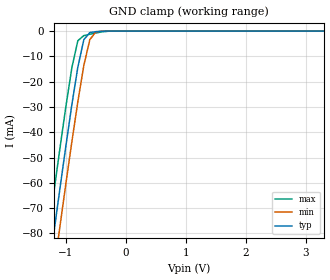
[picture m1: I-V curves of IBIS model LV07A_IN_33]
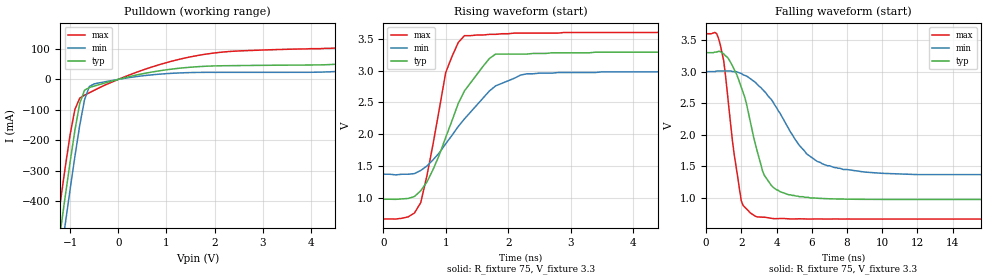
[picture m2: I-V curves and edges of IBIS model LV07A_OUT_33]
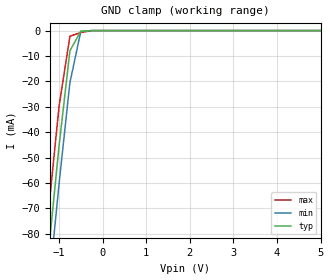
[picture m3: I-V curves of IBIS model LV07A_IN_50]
| TEXAS INSTRUMENTS INCORPORATED
| Standard Linear and Logic Group
| IBIS Model of SN74LV07A
| HEX BUFFER with OPEN DRAIN OUTPUTS
| SOIC 14-pin (D), SOP 14-pin (NS), SSOP 14-pin (DB), TSSOP 14-pin (PW)
| and TVSOP 14-pin (DGV) Package
[IBIS Ver]   3.2
[Comment Char]  |_char
[File Name]   sn74lv07a.ibs
[File Rev]   1.1
[Date]   July 27, 2004
[Source]   Data created from HSPICE simulations at TI-SLL.
[Notes]   The following is an IBIS list for the LV07A.
|   Please contact sllibis@ti.com with questions and
|   comments concerning SLL IBIS models.
   - FILE REV HISTORY
   - 1.1 Release IBIS file on 07/27/04
[Disclaimer] Property of Texas Instruments Incorporated.  Unauthorized
   reproduction and/or distribution is strictly prohibited.
   This product is protected under copyright law.
   Created  2004, (C) Copyright  2004, Texas Instruments
   Incorporated, All Rights Reserved
   UNLESS THERE IS A SIGNED, WRITTEN AGREEMENT TO THE
   CONTRARY, TEXAS INSTRUMENTS (TI) IS PROVIDING THE IBIS
   MODELS  AND WITHOUT ANY WARRANTY, EXPRESSED OR
   IMPLIED.  TI assumes no liability for:
   1) the accuracy of the IBIS models provided to your
   company;
   2) the proper functioning of these IBIS Models in your
   design or for any resulting applications; or
   3) infringement of patents, copyrights or intellectual
   property rights resulting from your use of these IBIS
   models.
   TI provides IBIS Models as a service to our customers.
   You and your company shall not distribute, sell or give
   these models to anyone else without prior written
   permission from TI.
   TI reserves the right to make changes to our products or
   to discontinue any semiconductor product or service
   without notice, and advises our customers to obtain the
   latest version of relevant information to verify, before
   placing orders, that the information being relied on is
   current.
   Please be aware that your receipt and use of the IBIS
   information provided shall serve as acceptance of these
   terms and conditions.  If you do not accept these terms,
   you should return or destroy the IBIS models and any
   other accompanying information immediately.
|   Component LV07A_D
[Component]   LV07A_D
[Manufacturer]  Texas Instruments, Inc.
[Package]
|   typ   min   max
R_pkg   0.031   0.028   0.034
L_pkg   3.109nH   2.462nH   3.889nH
C_pkg   0.473pF   0.363pF   0.628pF
[Pin]   signal_name   model_name   R_pin   L_pin   C_pin
1   1A   LV07A_IN   0.033   3.854nH   0.622pF
2   1Y   LV07A_OUT   0.032   3.188nH   0.473pF
3   2A   LV07A_IN   0.028   2.462nH   0.377pF
4   2Y   LV07A_OUT   0.031   2.596nH   0.363pF
5   3A   LV07A_IN   0.028   2.521nH   0.372pF
6   3Y   LV07A_OUT   0.034   3.250nH   0.476pF
7   GND   GND   0.034   3.889nH   0.628pF
8   4Y   LV07A_OUT   0.034   3.889nH   0.628pF
9   4A   LV07A_IN   0.034   3.250nH   0.476pF
10   5Y   LV07A_OUT   0.028   2.521nH   0.372pF
11   5A   LV07A_IN   0.031   2.596nH   0.364pF
12   6Y   LV07A_OUT   0.028   2.462nH   0.377pF
13   6A   LV07A_IN   0.032   3.188nH   0.473pF
14   VCC   POWER   0.033   3.854nH   0.622pF
|   Component LV07A_NS
[Component]   LV07A_NS
[Manufacturer]  Texas Instruments, Inc.
[Package]
|   typ   min   max
R_pkg   0.045   0.039   0.054
L_pkg   3.796nH   2.561nH   4.952nH
C_pkg   0.528pF   0.288pF   0.710pF
[Pin]   signal_name   model_name   R_pin   L_pin   C_pin
1   1A   LV07A_IN   0.047   4.867nH   0.706pF
2   1Y   LV07A_OUT   0.051   4.083nH   0.592pF
3   2A   LV07A_IN   0.041   2.915nH   0.376pF
4   2Y   LV07A_OUT   0.039   2.561nH   0.288pF
5   3A   LV07A_IN   0.041   3.101nH   0.430pF
6   3Y   LV07A_OUT   0.047   4.047nH   0.589pF
7   GND   GND   0.051   4.909nH   0.700pF
8   4Y   LV07A_OUT   0.045   4.784nH   0.694pF
9   4A   LV07A_IN   0.054   4.176nH   0.597pF
10   4Y   LV07A_OUT   0.039   3.287nH   0.449pF
11   5A   LV07A_IN   0.039   2.586nH   0.294pF
12   6Y   LV07A_OUT   0.040   2.802nH   0.371pF
13   6A   LV07A_IN   0.049   4.080nH   0.593pF
14   VCC   POWER   0.052   4.952nH   0.710pF
|   Component LV07A_DB
[Component]   LV07A_DB
[Manufacturer]  Texas Instruments, Inc.
[Package]
|   typ   min   max
R_pkg   0.044   0.041   0.046
L_pkg   3.551nH   3.258nH   3.927nH
C_pkg   0.402pF   0.360pF   0.421pF
[Pin]   signal_name   model_name   R_pin   L_pin   C_pin
1   1A   LV07A_IN   0.046   3.927nH   0.408pF
2   1Y   LV07A_OUT   0.044   3.587nH   0.421pF
3   2A   LV07A_IN   0.041   3.289nH   0.398pF
4   2Y   LV07A_OUT   0.042   3.258nH   0.360pF
5   3A   LV07A_IN   0.041   3.286nH   0.403pF
6   3Y   LV07A_OUT   0.044   3.586nH   0.421pF
7   GND   GND   0.046   3.927nH   0.408pF
8   4Y   LV07A_OUT   0.046   3.927nH   0.408pF
9   4A   LV07A_IN   0.044   3.586nH   0.421pF
10   5Y   LV07A_OUT   0.041   3.286nH   0.403pF
11   5A   LV07A_IN   0.043   3.258nH   0.360pF
12   6Y   LV07A_OUT   0.041   3.289nH   0.398pF
13   6A   LV07A_IN   0.044   3.587nH   0.421pF
14   VCC   POWER   0.046   3.927nH   0.408pF
|   Component LV07A_PW
[Component]   LV07A_PW
[Manufacturer]  Texas Instruments, Inc.
[Package]
|   typ   min   max
R_pkg   0.032   0.029   0.035
L_pkg   2.378nH   2.170nH   2.680nH
C_pkg   0.314pF   0.270pF   0.335pF
[Pin]   signal_name   model_name   R_pin   L_pin   C_pin
1   1A   LV07A_IN   0.033   2.618nH   0.330pF
2   1Y   LV07A_OUT   0.031   2.313nH   0.317pF
3   2A   LV07A_IN   0.030   2.310nH   0.314pF
4   2Y   LV07A_OUT   0.031   2.173nH   0.272pF
5   3A   LV07A_IN   0.030   2.204nH   0.309pF
6   3Y   LV07A_OUT   0.032   2.315nH   0.317pF
7   GND   GND   0.035   2.680nH   0.335pF
8   4Y   LV07A_OUT   0.033   2.640nH   0.333pF
9   4A   LV07A_IN   0.034   2.347nH   0.319pF
10   5Y   LV07A_OUT   0.029   2.277nH   0.313pF
11   5A   LV07A_IN   0.031   2.170nH   0.270pF
12   6Y   LV07A_OUT   0.031   2.244nH   0.311pF
13   6A   LV07A_IN   0.033   2.343nH   0.321pF
14   VCC   POWER   0.035   2.657nH   0.332pF
|   Component LV07A_DGV
[Component]   LV07A_DGV
[Manufacturer]  Texas Instruments, Inc.
[Package]
|   typ   min   max
R_pkg   0.035   0.020   0.045
L_pkg   2.499nH   2.077nH   2.966nH
C_pkg   0.361pF   0.305pF   0.416pF
[Pin]   signal_name   model_name   R_pin   L_pin   C_pin
1   1A   LV07A_IN   0.027   2.717nH   0.373pF
2   1Y   LV07A_OUT   0.037   2.434nH   0.398pF
3   2A   LV07A_IN   0.034   2.200nH   0.316pF
4   2Y   LV07A_OUT   0.020   2.077nH   0.309pF
5   3A   LV07A_IN   0.030   2.147nH   0.305pF
6   3Y   LV07A_OUT   0.042   2.580nH   0.408pF
7   GND   GND   0.039   2.921nH   0.385pF
8   4Y   LV07A_OUT   0.033   2.841nH   0.380pF
9   4A   LV07A_IN   0.042   2.611nH   0.410pF
10   5Y   LV07A_OUT   0.038   2.331nH   0.329pF
11   5A   LV07A_IN   0.026   2.223nH   0.319pF
12   6Y   LV07A_OUT   0.034   2.259nH   0.313pF
13   6A   LV07A_IN   0.045   2.681nH   0.416pF
14   VCC   POWER   0.042   2.966nH   0.386pF
[Model Selector]   LV07A_IN
LV07A_IN_33   3.3-V Vcc Input Model
LV07A_IN_50   5.0-V Vcc Input Model
[Model Selector]   LV07A_OUT
LV07A_OUT_33   3.3-V Vcc Output Model
LV07A_OUT_50   5.0-V Vcc Output Model
| Models and submodels in the file (4): LV07A_IN_33 (Input), LV07A_OUT_33 (Open_drain), LV07A_IN_50 (Input), LV07A_OUT_50 (Open_drain)
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|   Model LV07A_IN_33
[Model]   LV07A_IN_33
Model_type  Input
Polarity   Non-Inverting
Vinl = 0.99
Vinh = 2.31
| variable   typ   min   max
C_comp   1.24pf   0.94pf   1.54pf
[Temperature Range]   25   85   -40
[Voltage Range]   3.3   3.0   3.6
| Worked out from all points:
|   GND clamp passes 1 mA (typ) near -0.61 V on its own axis
[GND Clamp]
|   Voltage   I(typ)   I(min)   I(max)
-3.3V     -460mA     -475mA     -445mA
-1.3V     -97.5mA    -113mA     -81.5mA
-1.2V     -79.9mA    -95mA      -63.9mA
-1.1V     -62.6mA    -77.6mA    -46.7mA
-1V       -45.6mA    -60.5mA    -30mA
-900mV    -29.2mA    -43.9mA    -14.6mA
-800mV    -14.3mA    -28mA      -3.81mA
-700mV    -3.42mA    -13.6mA    -1.78mA
-600mV    -581uA     -3.4mA     -1.25mA
-500mV    -233uA     -353uA     -759uA
-400mV    -58.1uA    -21.9uA    -324uA
3.3V      1.9nA      2.34nA     1.69nA
|   Model LV07A_OUT_33
[Model]   LV07A_OUT_33
Model_type  Open_drain
Polarity   Non-Inverting
Vmeas = 1.65v
Cref = 15pf
| variable   typ   min   max
C_comp   4.62pf   3.47pf   5.77pf
[Temperature Range]   25   85   -40
[Voltage Range]   3.3   3.0   3.6
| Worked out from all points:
|   slope of the pulldown table from 0 to 0.495 V, typ, clamps not added: 27.3 ohm
|   falling waveform, R_fixture 75, V_fixture 3.3: 20-80 % time 1.3ns typ, 2.37ns min, 767ps max; typ from 3.3 V to 0.976 V
|   rising waveform, R_fixture 75, V_fixture 3.3: 20-80 % time 624ps typ, 807ps min, 340ps max; typ from 0.976 V to 3.3 V
[Pulldown]
|   Voltage   I(typ)   I(min)   I(max)
-3.3V     -3.04A     -3.13A     -2.95A
-1.3V     -615mA     -707mA     -518mA
-1.2V     -498mA     -591mA     -401mA
-1.1V     -383mA     -475mA     -288mA
-900mV    -167mA     -253mA     -98.6mA
-800mV    -79.1mA    -151mA     -61.7mA
-700mV    -35.5mA    -66.4mA    -51.9mA
-600mV    -26.8mA    -23.2mA    -43.9mA
-500mV    -22mA      -14.7mA    -35.8mA
1.6V      41.2mA     22.8mA     77.1mA
4.7V      52.1mA     27.5mA     106mA
6.6V      86.8mA     47.3mA     166mA
[Ramp]
| variable   typ   min   max
dV/dt_r   1.40E+00/1.34E-09   9.37E-01/2.69E-09   1.78E+00/5.88E-10
dV/dt_f   1.41E+00/1.30E-09   9.88E-01/2.40E-09   1.77E+00/7.47E-10
R_load = 75
[Falling Waveform]
R_fixture = 75
V_fixture = 3.3
V_fixture_min = 3.0
V_fixture_max = 3.6
|   Time   V(typ)   V(min)   V(max)
0s        3.3V       3V         3.6V
800ps     3.32V      3.01V      3.43V
1ns       3.28V      3.01V      3.17V
2ns       2.75V      2.97V      951mV
2.8ns     1.85V      2.83V      710mV
3.3ns     1.36V      2.69V      695mV
4ns       1.13V      2.43V      673mV
5.7ns     1.01V      1.7V       667mV
7.3ns     985mV      1.48V      667mV
25ns      976mV      1.37V      666mV
[Rising Waveform]
R_fixture = 75
V_fixture = 3.3
V_fixture_min = 3.0
V_fixture_max = 3.6
|   Time   V(typ)   V(min)   V(max)
0s        976mV      1.37V      666mV
400ps     989mV      1.37V      700mV
600ps     1.11V      1.43V      924mV
800ps     1.45V      1.6V       1.86V
1ns       1.95V      1.85V      2.97V
1.3ns     2.68V      2.24V      3.55V
1.8ns     3.26V      2.76V      3.57V
2.2ns     3.26V      2.93V      3.59V
2.8ns     3.28V      2.97V      3.59V
25ns      3.3V       3V         3.6V
|   Model LV07A_IN_50
[Model]   LV07A_IN_50
Model_type  Input
Polarity   Non-Inverting
Vinl = 1.5
Vinh = 3.5
| variable   typ   min   max
C_comp   1.24pf   0.94pf   1.54pf
[Temperature Range]   25   85   -40
[Voltage Range]   5.0   4.5   5.5
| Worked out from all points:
|   GND clamp passes 1 mA (typ) near -0.52 V on its own axis
[GND Clamp]
|   Voltage   I(typ)   I(min)   I(max)
-5V       -773mA     -786mA     -758mA
-1.5V     -133mA     -148mA     -117mA
-1.25V    -88.7mA    -104mA     -72.7mA
-1V       -45.6mA    -60.5mA    -30mA
-750mV    -7.99mA    -20.5mA    -2.23mA
-500mV    -233uA     -353uA     -759uA
-250mV    -2.63nA    -182nA     -26.9uA
5V        2.9nA      3.64nA     2.54nA
